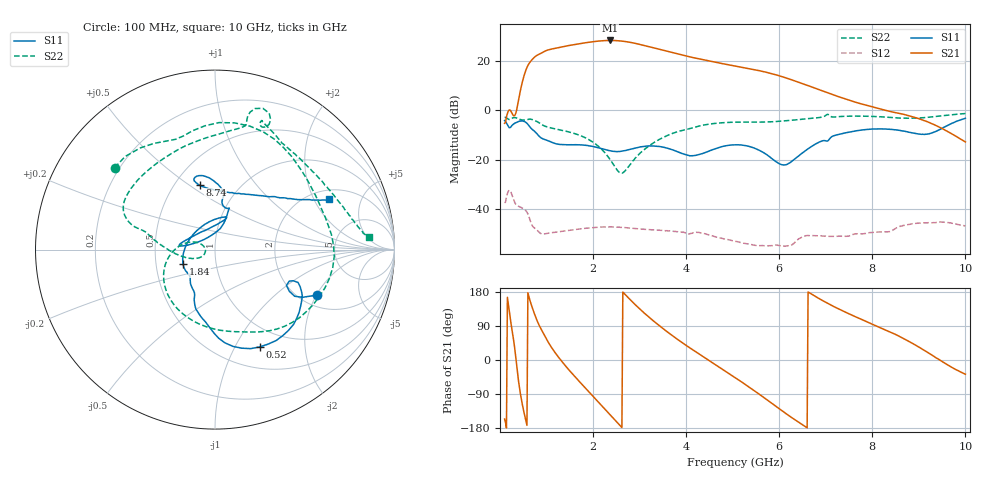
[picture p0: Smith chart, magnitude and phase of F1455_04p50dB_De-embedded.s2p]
! Integrated Device Technology
! Corporate Headquarters
! 6024 Silver Creek Valley Road
! San Jose, CA 95138  USA
! Phone:  1-408-284-8200
! Toll Free:  1-800-223-1366
! Webpage:  http://www.idt.com/
! Timing and RF Division
! 515 Groton Road, Suite 102
! Westford, MA 01886-6024
! Device:  F1455
! Description: 6-bit 0.5 dB Transmit Variable Gain Amplifier
! Frequency:  1400.0 -  2300.00 MHz
! Package:  6x6 mm Thin QFN Plastic Package: 28 pin
! State:  9
! Atten State:  4.5 dB
! Voltage:  +5.00 Volts
! Current:  216.084 mA
! Data:  The device was measured on a the F1455 evaluation board which has
!  individual transmission lines to the RF pins.  Data was collected
!  using a calibrated network analyzer.  The evaluation board was
!  de-embedded using a TRL calibration technique.
!  The reference plane is the edge of the package pin.
!  Pin  1 = CSb
!  Pin  2 = DATA
!  Pin  3 = CLK
!  Pin  4 = RSET
!  Pin  5 = GND
!  Pin  6 = RFIN  = Port 1
!  Pin  7 = GND
!  Pin  8 = NC
!  Pin  9 = NC
!  Pin 10 = NC
!  Pin 11 = NC
!  Pin 12 = NC
!  Pin 13 = NC
!  Pin 14 = /STBY
!  Pin 15 = GND
!  Pin 16 = RFOUT  = Port 2
!  Pin 17 = GND
!  Pin 18 = NC
!  Pin 19 = NC
!  Pin 20 = NC
!  Pin 21 = GND
!  Pin 22 = NC
!  Pin 23 = GND
!  Pin 24 = NC
!  Pin 25 = NC
!  Pin 26 = NC
!  Pin 27 = GND
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# GHz S dB R 50
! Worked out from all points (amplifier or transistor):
!   496 points, 100 MHz to 10 GHz, reference 50 ohm
!   highest |S21| = 28.3 dB at 2.36 GHz (marker M1)
!   |S21| within 3 dB of that: 1.228 GHz to 3.305 GHz (2.077 GHz wide, 91.7 % of centre)
!   unconditionally stable (mu >= 1): start of sweep to end of sweep
!   at 1.74 GHz: K = 4.83, MAG = 27.7 dB, |S12| = -48.0 dB
!   at 5.06 GHz: K = 18.24, MAG = 19.9 dB, |S12| = -53.0 dB
!   at 10 GHz: K = 63.42, MAG = -4.0 dB, |S12| = -46.8 dB
!   S11 on the Smith chart (normalised r, x): 100 MHz: 2.42, -2.01; 520 MHz: 0.75, -1.26; 1.84 GHz: 0.69, -0.12; 8.74 GHz: 0.66, +0.55; 10 GHz: 2.45, +2.63
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0.1  -4.14 -24.3  -5.24 -155.8  -37.48 41.2  -2.83 140.8
0.38  -4.66 -36.8  2.14 -36.8  -38.67 -107.9  -3.30 55.9
0.52  -4.49 -65.3  14.18 -140.3  -40.03 -152.7  -3.94 24.3
0.7  -7.82 -97.4  20.74 136.0  -46.83 152.0  -3.76 -19.4
0.82  -10.05 -111.4  22.53 97.4  -48.97 135.7  -4.78 -47.9
0.96  -11.80 -117.8  23.92 64.2  -50.00 124.3  -6.35 -72.2
1.14  -13.12 -128.8  24.95 27.2  -49.45 102.0  -7.30 -96.9
1.34  -13.88 -134.8  25.74 -5.4  -48.96 80.1  -8.11 -120.7
1.76  -13.99 -150.8  27.15 -64.0  -47.89 45.1  -10.45 -159.9
1.84  -14.14 -155.2  27.39 -74.5  -47.77 39.2  -11.15 -166.6
2.1  -15.06 -173.8  28.02 -108.7  -47.33 21.7  -14.31 172.8
2.36  -16.35 156.3  28.31 -143.6  -47.16 5.1  -19.71 158.0
2.62  -16.53 117.6  28.05 -178.1  -47.38 -10.3  -25.44 -173.4
2.92  -15.17 85.3  27.08 144.4  -47.86 -25.0  -19.08 -154.4
3.4  -14.56 70.1  24.85 92.9  -48.52 -44.4  -12.04 -178.5
4.08  -18.39 109.1  21.66 31.9  -49.99 -68.3  -7.36 164.8
5.06  -13.91 172.9  17.95 -47.0  -53.04 -105.7  -4.78 148.9
5.94  -20.87 146.8  14.35 -123.3  -54.53 -115.5  -4.50 109.2
6.7  -14.55 70.9  9.48 173.5  -50.70 -140.8  -3.20 78.4
8.36  -7.64 106.0  -0.35 74.9  -49.12 165.5  -2.82 62.4
8.74  -8.63 103.5  -1.95 52.1  -46.31 153.9  -3.19 48.9
10  -3.19 23.8  -12.77 -37.6  -46.82 80.6  -1.30 4.6
